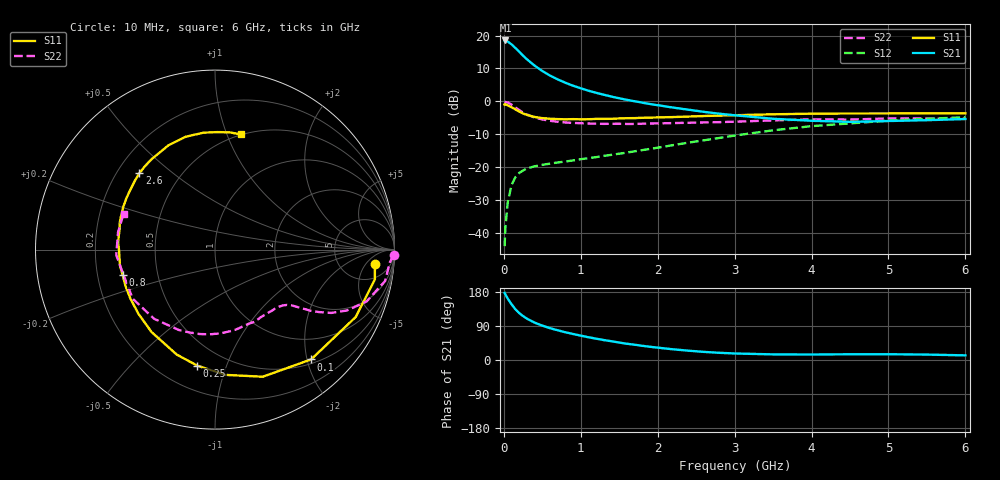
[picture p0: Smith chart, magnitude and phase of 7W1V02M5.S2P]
! Infineon Technologies  Discrete & RF Semiconductors
! BFS17W
! Si NPN RF Bipolar Junction Transistor in SOT323
! VCE = 1 V  IC = 2.5 mA
! Common Emitter S-Parameters:  August  1999
# GHz  S  MA  R  50
!  f  S11  S21  S12  S22
! GHz  MAG  ANG  MAG  ANG  MAG  ANG  MAG  ANG
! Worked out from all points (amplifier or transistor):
!   36 points, 10 MHz to 6 GHz, reference 50 ohm
!   highest |S21| = 18.5 dB at 20 MHz (marker M1)
!   |S21| within 3 dB of that: start of sweep to 181.1 MHz
!   unconditionally stable (mu >= 1): 691 MHz to end of sweep
!   at 250 MHz: K = 0.43, MSG = 17.4 dB, |S12| = -21.0 dB
!   at 1.4 GHz: K = 1.38, MAG = 5.2 dB, |S12| = -16.3 dB
!   at 6 GHz: K = 1.13, MAG = -2.5 dB, |S12| = -4.8 dB
!   S11 on the Smith chart (normalised r, x): 10 MHz: 11, -9; 100 MHz: 0.57, -2.07; 250 MHz: 0.35, -0.80; 800 MHz: 0.31, -0.12; 2.6 GHz: 0.29, +0.39; 6 GHz: 0.49, +1.12
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0.01  0.8946 -5.2  8.355 177.1  0.0063 84.3  0.995 -1.7
0.02  0.9062 -10.6  8.428 172.9  0.012 85.8  0.9767 -4.2
0.05  0.8692 -25.6  8.106 162.3  0.029 76.8  0.9642 -10.4
0.1  0.8132 -48.8  7.352 147.0  0.0534 64.3  0.8927 -18.9
0.15  0.7567 -69.4  6.483 133.9  0.0705 54.9  0.8091 -24.8
0.2  0.7001 -85.4  5.673 123.8  0.0818 48.8  0.7371 -28.6
0.25  0.6539 -98.7  4.947 115.8  0.0891 44.0  0.6754 -31.0
0.3  0.6226 -110.0  4.36 109.1  0.0955 41.1  0.6322 -32.6
0.4  0.5796 -127.6  3.496 98.6  0.1031 37.5  0.5673 -34.6
0.5  0.5565 -140.1  2.895 90.7  0.1085 36.4  0.5314 -35.9
0.6  0.5445 -150.1  2.467 84.0  0.1132 36.4  0.506 -37.5
0.8  0.5338 -164.7  1.92 73.2  0.122 38.2  0.4782 -41.7
0.9  0.5371 -170.4  1.729 68.6  0.1266 39.3  0.4695 -44.0
1.1  0.5353 179.7  1.453 60.0  0.137 42.0  0.4609 -49.5
1.3  0.5419 171.4  1.261 52.6  0.1485 44.3  0.4548 -55.8
1.6  0.5549 161.4  1.054 42.9  0.1666 47.6  0.4536 -65.5
2.2  0.5774 144.9  0.805 28.2  0.2163 52.2  0.4679 -86.3
2.6  0.599 134.7  0.693 21.4  0.2561 52.9  0.4783 -100.5
3.5  0.6363 114.1  0.544 14.8  0.3631 48.7  0.5136 -131.4
4.5  0.6546 95.6  0.488 15.1  0.4628 37.5  0.5285 -164.3
5.5  0.6583 82.6  0.518 14.3  0.5422 26.6  0.5487 169.9
6  0.6574 77.5  0.539 12.2  0.5741 21.3  0.5475 158.5
